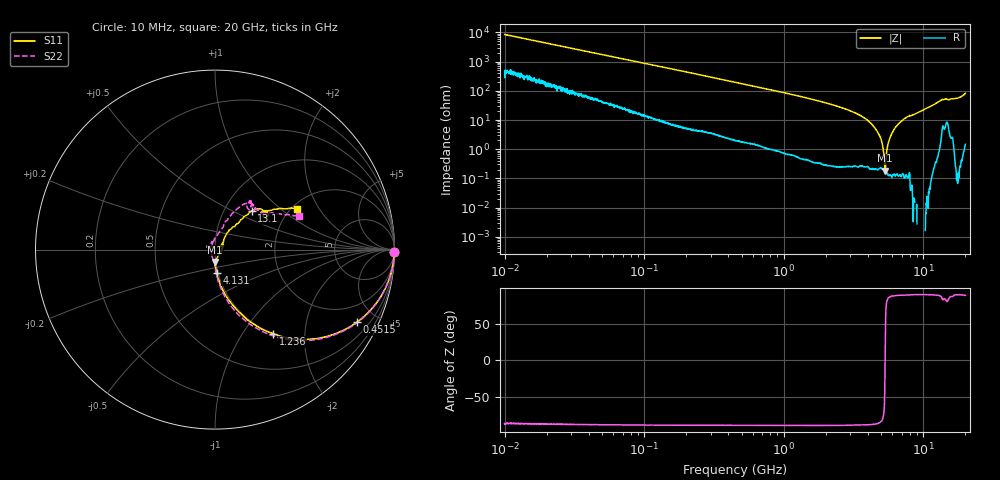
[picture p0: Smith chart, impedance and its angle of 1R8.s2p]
!Keysight Technologies,P5008B,MY61100088,A.16.20.02
!Date: Friday, August 30, 2024 11:04:54
!Correction: S11(C  2-Port  )
!S21(C  2-Port  )
!S12(C  2-Port  )
!S22(C  2-Port  )
!S2P File: Measurements: S11, S21, S12, S22:Log Frequency Sweep
# Hz S  dB  R 50
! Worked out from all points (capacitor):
!   1601 points, 10 MHz to 20 GHz, reference 50 ohm
!   read as one part in series: C = 1.87 pF near 10.39 MHz
!   lowest |Z| = 182 mohm at 5.314 GHz (marker M1)
!   series resonance near 5.321 GHz, so ESL is about 480 pH
!   S11 on the Smith chart (normalised r, x): 10 MHz: open; 451.5 MHz: 1.02, -3.89; 1.236 GHz: 1.00, -1.39; 4.131 GHz: 0.98, -0.26; 13.1 GHz: 1.34, +0.64; 20 GHz: 2.13, +1.31
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1e7  -0.00 -0.7  -38.60 86.7  -38.59 86.7  -0.01 -0.7
3.555162e7  -0.02 -2.4  -27.75 85.9  -27.75 85.9  -0.02 -2.4
1.263918e8  -0.11 -8.2  -16.98 80.9  -16.98 80.9  -0.10 -8.4
2.57745e8  -0.38 -16.3  -11.13 72.9  -11.13 72.9  -0.38 -16.6
4.472136e8  -1.02 -26.9  -6.97 62.3  -6.97 62.3  -1.02 -27.4
4.514829e8  -1.04 -27.2  -6.90 62.0  -6.90 62.0  -1.04 -27.6
7.759606e8  -2.53 -41.6  -3.64 47.5  -3.64 47.5  -2.53 -42.3
1.236026e9  -4.87 -55.3  -1.76 33.5  -1.76 33.5  -4.88 -56.8
1.589917e9  -6.63 -62.7  -1.09 26.1  -1.10 26.1  -6.63 -64.3
2.824976e9  -11.96 -77.6  -0.31 11.1  -0.31 11.1  -11.93 -79.0
4.131105e9  -17.83 -86.0  -0.09 2.1  -0.09 2.1  -17.80 -87.5
5.313894e9  -23.22 -89.6  -0.03 -3.9  -0.03 -3.9  -23.43 -93.5
5.652411e9  -24.64 -86.2  -0.01 -5.4  -0.02 -5.4  -25.10 -99.9
6.643251e9  -29.58 -37.3  0.01 -9.4  0.00 -9.4  -31.78 -159.7
7.697294e9  -27.15 27.0  0.01 -13.3  0.01 -13.4  -28.36 119.1
8.344716e9  -28.59 30.1  0.02 -15.5  0.02 -15.6  -29.53 110.7
1.104427e10  -17.81 53.5  -0.03 -25.6  -0.03 -25.6  -18.03 71.6
1.310419e10  -10.52 46.4  -0.41 -34.4  -0.42 -34.5  -10.68 58.5
1.407205e10  -9.35 38.5  -0.79 -36.4  -0.80 -36.5  -9.97 50.7
1.709804e10  -9.51 38.5  -0.47 -44.9  -0.47 -45.0  -9.68 49.9
1.836088e10  -9.18 37.8  -0.52 -52.1  -0.52 -52.3  -9.30 36.3
2e10  -5.86 26.5  -1.36 -64.2  -1.36 -64.3  -5.93 21.7
